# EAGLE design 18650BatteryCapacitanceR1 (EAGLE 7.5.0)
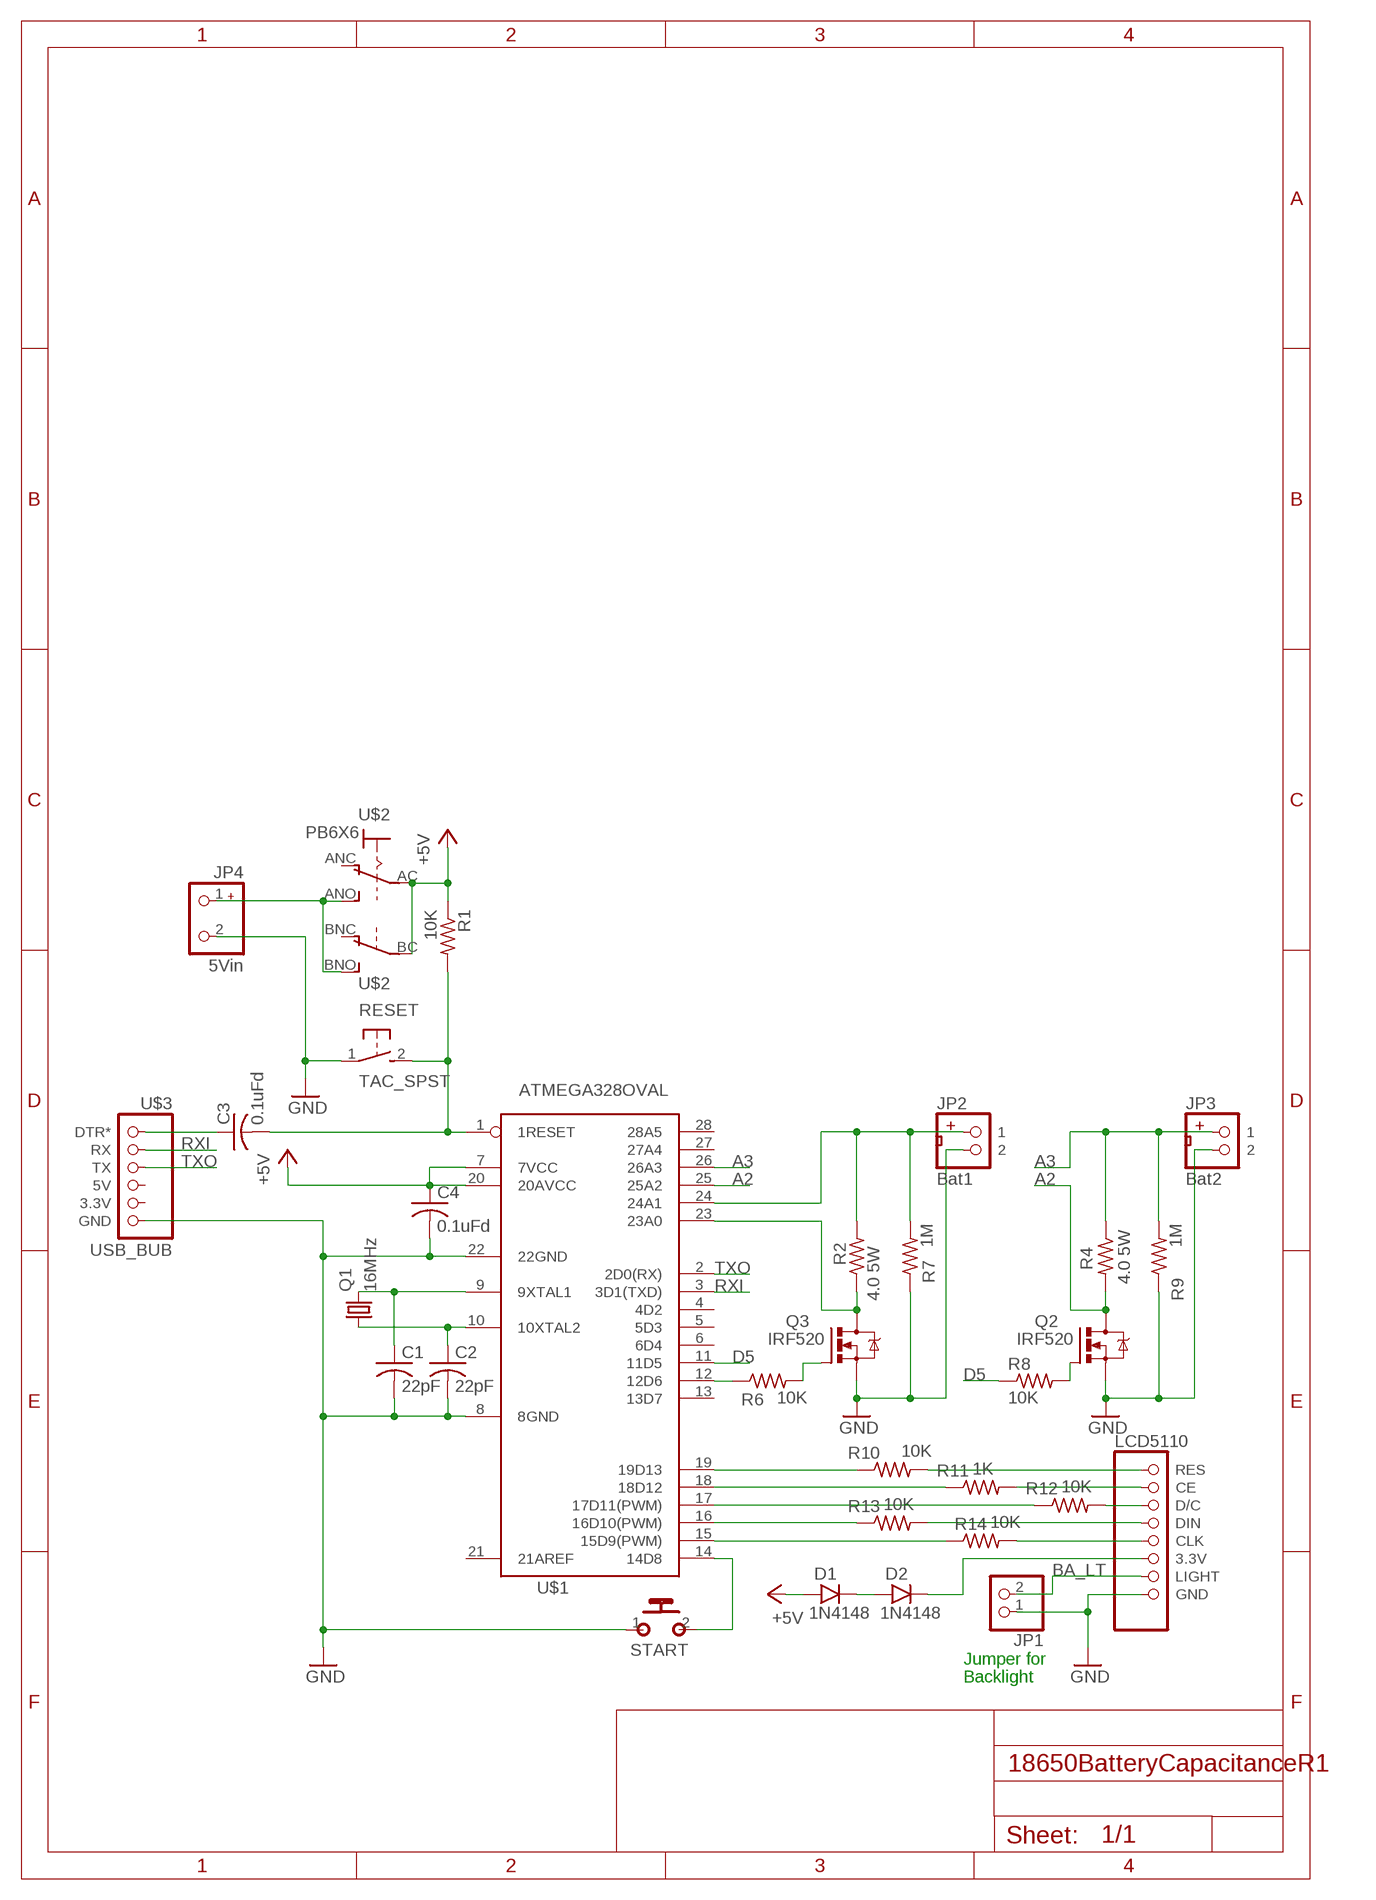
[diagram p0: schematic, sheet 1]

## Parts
C1  22pF  C-US025-025X050  [C025-025X050]
C2  22pF  C-US025-025X050  [C025-025X050]
C3  0.1uFd  C-US075-032X103  [C075-032X103]
C4  0.1uFd  C-US025-025X050  [C025-025X050]
D1  1N4148  1N4148-3  [DO35-3]
D2  1N4148  1N4148-3  [DO35-3]
JP1  PINHD-1X2  [1X02]
JP2  Bat1  JST2.0  [JST2.0]
JP3  Bat2  JST2.0  [JST2.0]
JP4  5Vin  KF301  [KF301]
LCD5110  LCD5110_1TOP  [LCD5110T1]
Q1  16MHz  CRYSTALHC49S  [HC49/S]
Q2  IRF520  [TO220BV]
Q3  IRF520  [TO220BV]
R1  10K  R-US_0207/7  [0207/7]
R2  4.0 5W  R-US_0922/22  [0922/22]
R4  4.0 5W  R-US_0922/22  [0922/22]
R6  10K  R-US_0207/7  [0207/7]
R7  1M  R-US_0207/2V  [0207/2V]
R8  10K  R-US_0207/7  [0207/7]
R9  1M  R-US_0207/2V  [0207/2V]
R10  10K  R-US_0207/2V  [0207/2V]
R11  1K  R-US_0207/2V  [0207/2V]
R12  10K  R-US_0207/2V  [0207/2V]
R13  10K  R-US_0207/2V  [0207/2V]
R14  10K  R-US_0207/2V  [0207/2V]
RESET  TAC_SPST  [TACTILE-SPST]
START  MOMENTARY  [SPST]
U$1  ATMEGA328OVAL  [DIL28-3]
U$2  PB6X6  [PB6X6]
U$3  USB_BUB  [USB_BUB]

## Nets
+5V: C4.1 D1.A R1.1 U$1.7(7VCC) U$1.20(20AVCC) U$2.AC(P) U$2.BC(P)
A2: Q2.D R4.2 U$1.25(25A2)
A3: JP3.1 R4.1 R9.2 U$1.26(26A3)
BA_LT: JP1.2 LCD5110.LIGHT
D5: R8.1 U$1.11(11D5)
GND: C1.2 C2.2 C4.2 JP1.1 JP2.2 JP3.2 JP4.2 LCD5110.GND Q2.S Q3.S R7.1 R9.1 RESET.1 START.1(P) U$1.8(8GND) U$1.22(22GND) U$3.GND
N$1: C1.1 Q1.2 U$1.9(9XTAL1)
N$2: C2.1 Q1.1 U$1.10(10XTAL2)
N$3: D2.C LCD5110.3.3V
N$4: JP4.1 U$2.ANO(S) U$2.BNO(S)
N$5: START.2(S) U$1.14(14D8)
N$6: C3.2 R1.2 RESET.2 U$1.1(1RESET)
N$7: C3.1 U$3.DTR*
N$8: Q2.G R8.2
N$9: D1.C D2.A
N$10: R10.1 U$1.19(19D13)
N$11: R11.1 U$1.18(18D12)
N$12: R12.1 U$1.17(17D11(PWM))
N$13: R13.1 U$1.16(16D10(PWM))
N$14: R14.1 U$1.15(15D9(PWM))
N$15: R6.1 U$1.12(12D6)
N$16: Q3.G R6.2
N$18: Q3.D R2.1 U$1.23(23A0)
N$20: JP2.1 R2.2 R7.2 U$1.24(24A1)
N$24: LCD5110.RES R10.2
N$25: LCD5110.CE R11.2
N$26: LCD5110.D/C R12.2
N$27: LCD5110.DIN R13.2
N$28: LCD5110.CLK R14.2
RXI: U$1.3(3D1(TXD)) U$3.RX
TXO: U$1.2(2D0(RX)) U$3.TX
Unconnected: U$1.4(4D2) U$1.5(5D3) U$1.6(6D4) U$1.13(13D7) U$1.21(21AREF) U$1.27(27A4) U$1.28(28A5) U$2.ANC(O) U$2.BNC(O) U$3.3.3V U$3.5V

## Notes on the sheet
- Jumper for
- Backlight

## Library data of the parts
C1-C4 = rcl:C-US: CAPACITOR, American symbol
D1 D2 = gm-diodes:1N4148: Fast Switching Diode
JP1 = pinhead:PINHD-1X2: PIN HEADER
JP2 JP3 = MTS_Custom:JST2.0
JP4 = MTS_Custom:KF301
LCD5110 = MTS_Custom:LCD5110_1
Q1 = crystal:CRYSTAL: CRYSTAL; OC_FARNELL: 1667008; OC_NEWARK: unknown
Q2 Q3 = transistor-power:IRF520: HEXFET Power MOSFET
R1 R6-R14 = rcl:R-US_: RESISTOR, American symbol
R2 R4 = resistor:R-US_: RESISTOR, American symbol
RESET = MTS_Custom:TAC_SPST: Tactile switch SPST 7mm lead spacing
START = MTS_Custom:MOMENTARY
U$1 = MTS_Custom:ATMEGA328
U$2 = MTS_Custom:PB6X6: Pushbutton 6mm x 6mm DPDT. should be the same for momentary and latching.
U$3 = MTS:USB_BUB

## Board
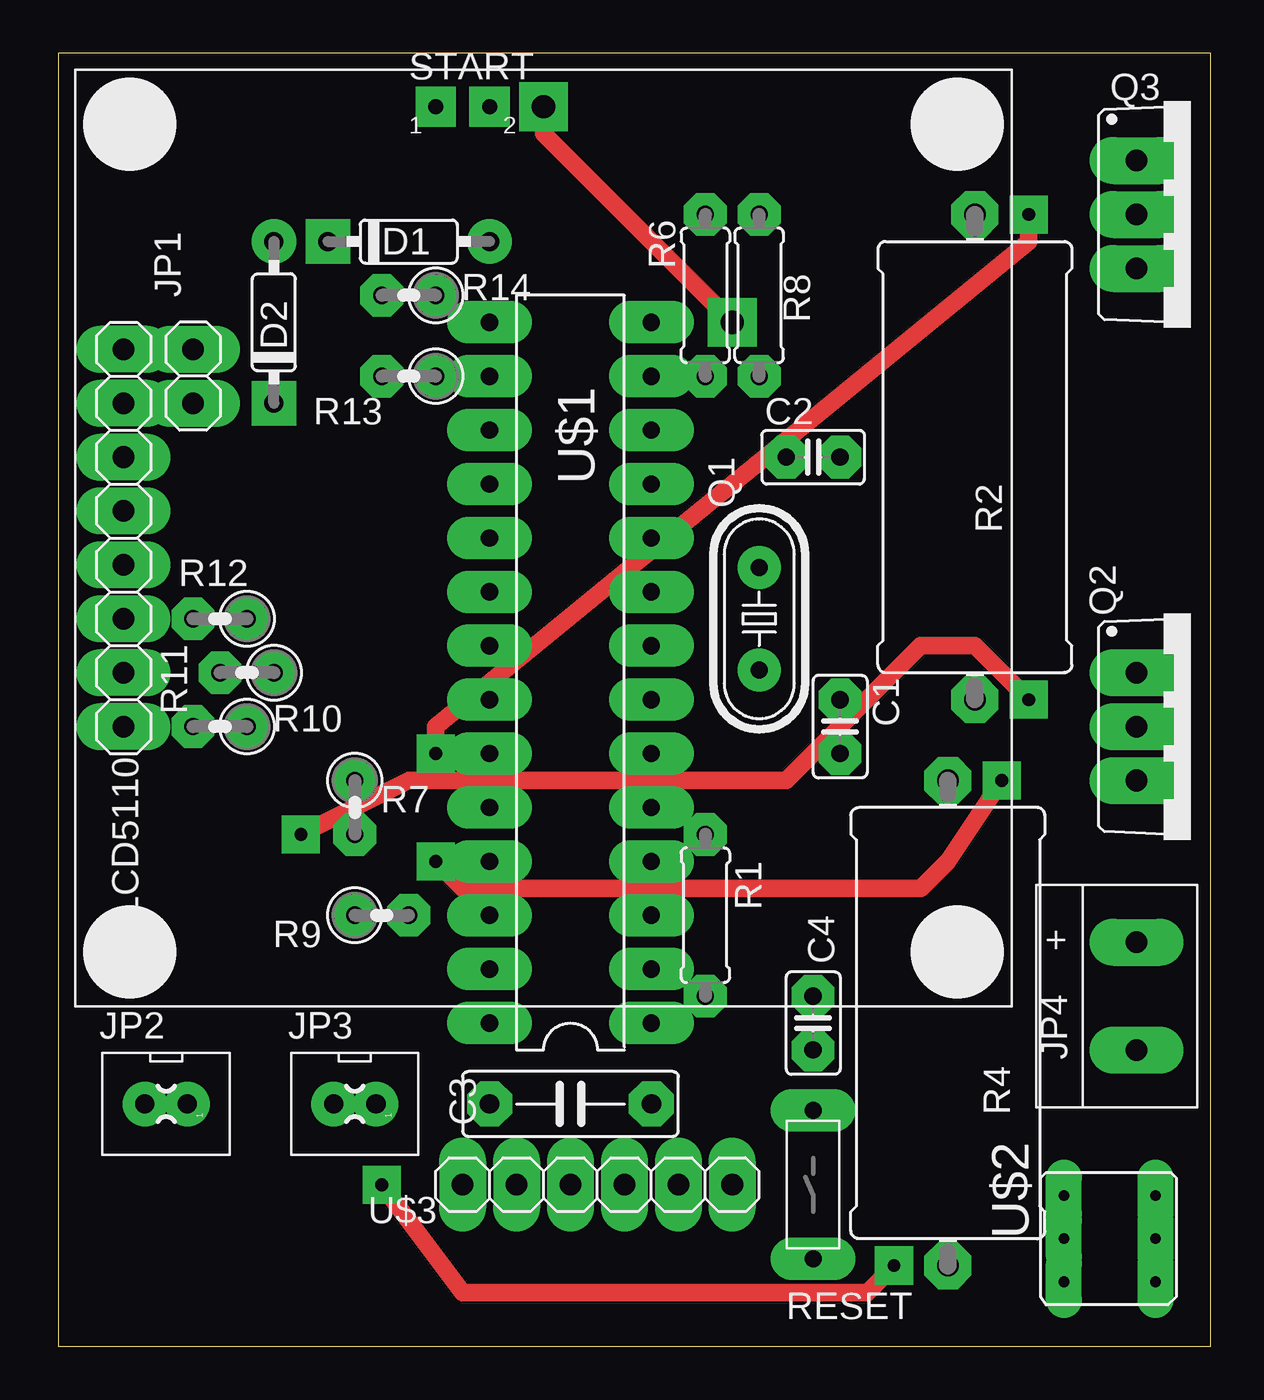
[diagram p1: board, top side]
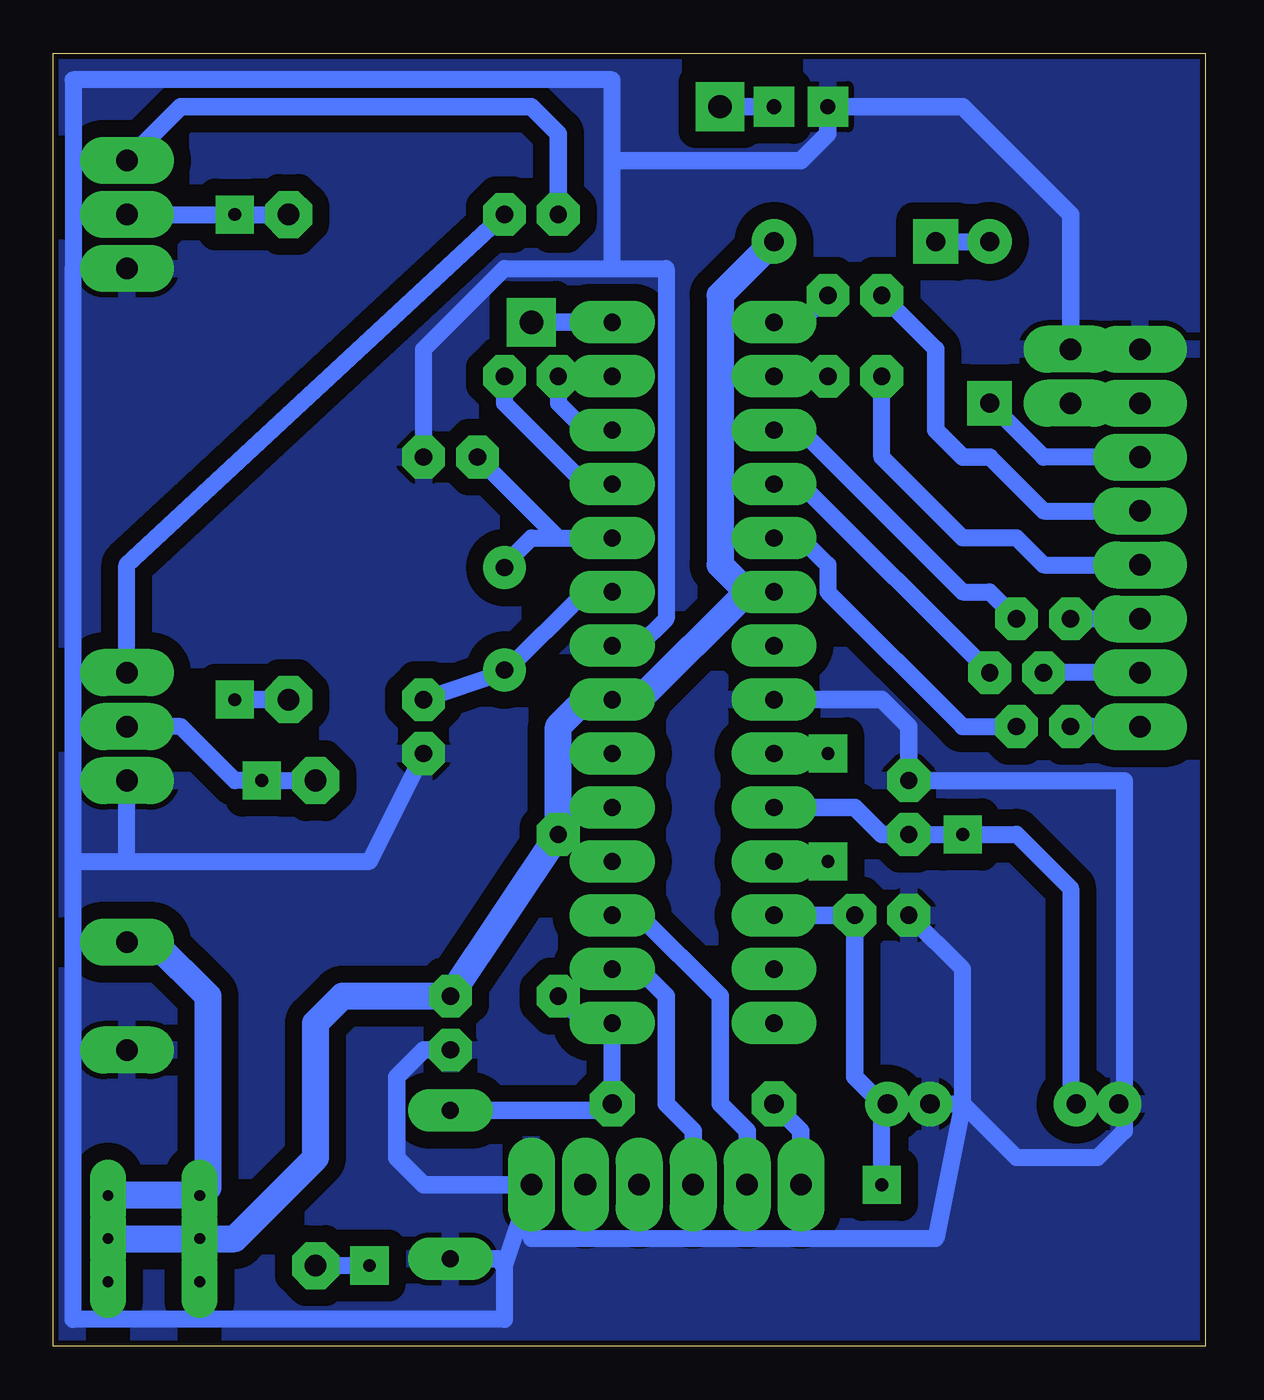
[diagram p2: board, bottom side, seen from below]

Size 54.28 x 60.95 mm. Coordinates in mm from the lower left corner, seen from the top.
Outline: 0,0 54.28,0 54.28,60.95 0,60.95 0,0
Copper layers (1*16): Top 0.035mm / dielectric 1.5mm / Bottom 0.035mm
Design rules "hobby": minimum track width 0.8mm, minimum drill 0.8mm, track to track 0.8mm, track to pad 0.8mm, pad to pad 0.45mm, via to via 0.8mm, smd to smd 8mil, copper to edge 10mil, drill to drill 8mil, minimum pad ring 0.6mm, minimum via ring 0.6mm, stop-mask expansion 0mil, vias tented up to drill 0mil, thermal gap 10mil

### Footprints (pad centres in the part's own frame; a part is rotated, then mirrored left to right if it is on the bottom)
C025-025X050 = drill 0.813 octagon: 1 -1.27,0; 2 1.27,0
C075-032X103 = drill 0.914 octagon: 1 -3.81,0; 2 3.81,0
DO35-3 = drill 0.9: A 3.81,0 | drill 0.9 square: C -3.81,0
1X02 = drill 1.016 long: 1 -1.27,0; 2 1.27,0
JST2.0 = drill 0.9 pad 1.016: 1 0,-1; 2 0,1
KF301 = drill 1.016 long: 1 -2.54,0; 2 2.54,0
LCD5110T1 = drill 1.016 long: 3.3V 3.81,19.78; CE -6.35,19.78; CLK 1.27,19.78; D/C -3.81,19.78; DIN -1.27,19.78; GND 8.89,19.78; LIGHT 6.35,19.78; RES -8.89,19.78
HC49/S = drill 0.813: 1 -2.413,0; 2 2.413,0
TO220BV = drill 1.016 long: D 0,-2.54; G -2.54,-2.54; S 2.54,-2.54
0207/7 = drill 0.813 octagon: 1 -3.81,0; 2 3.81,0
0922/22 = drill 1.016 octagon: 1 -11.43,0; 2 11.43,0
0207/2V = drill 0.813 octagon: 1 -1.27,0; 2 1.27,0
TACTILE-SPST = drill 0.8 long: 1 0,3.5; 2 0,-3.5
SPST = drill 0.7 square: 1 -1.27,0; 2 1.27,0
DIL28-3 = drill 0.813 long: 1 -16.51,-3.81; 2 -13.97,-3.81; 3 -11.43,-3.81; 4 -8.89,-3.81; 5 -6.35,-3.81; 6 -3.81,-3.81; 7 -1.27,-3.81; 8 1.27,-3.81; 9 3.81,-3.81; 10 6.35,-3.81; 11 8.89,-3.81; 12 11.43,-3.81; 13 13.97,-3.81; 14 16.51,-3.81; 15 16.51,3.81; 16 13.97,3.81; 17 11.43,3.81; 18 8.89,3.81; 19 6.35,3.81; 20 3.81,3.81; 21 1.27,3.81; 22 -1.27,3.81; 23 -3.81,3.81; 24 -6.35,3.81; 25 -8.89,3.81; 26 -11.43,3.81; 27 -13.97,3.81; 28 -16.51,3.81
PB6X6 = drill 0.5 pad 0.813 long: AC -2.159,0; ANC -2.159,-2.032; ANO -2.159,2.032; BC 2.159,0; BNC 2.159,-2.032; BNO 2.159,2.032
USB_BUB = drill 1.016 long: 3.3V -3.81,0; 5V -1.27,0; DTR* 6.35,0; GND -6.35,0; RX 3.81,0; TX 1.27,0

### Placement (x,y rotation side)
C1  36.83,29.21 270 top
C2  35.56,41.91 0 top
C3  24.13,11.43 0 top
C4  35.56,15.24 270 top
D1  16.51,52.07 0 top
D2  10.16,48.26 90 top
JP1  6.35,45.72 270 top
JP2  5.08,11.43 90 top
JP3  13.97,11.43 90 top
JP4  50.8,16.51 270 top
LCD5110  22.86,38.1 90 top
Q1  33.02,34.29 270 top
Q2  53.34,29.21 270 top
Q3  53.34,53.34 270 top
R1  30.48,20.32 270 top
R2  43.18,41.91 270 top
R4  41.91,15.24 90 top
R6  30.48,49.53 90 top
R7  13.97,25.4 270 top
R8  33.02,49.53 90 top
R9  15.24,20.32 0 top
R10  7.62,29.21 180 top
R11  8.89,31.75 180 top
R12  7.62,34.29 180 top
R13  16.51,45.72 180 top
R14  16.51,49.53 180 top
RESET  35.56,7.62 180 top
START  19.05,58.42 0 top
U$1  24.13,31.75 90 top
U$2  49.53,5.08 0 top
U$3  25.4,7.62 180 top

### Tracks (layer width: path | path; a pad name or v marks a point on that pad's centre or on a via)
+5V
  Bottom 1.27: 21.59,35.56 U$1.20 | 21.59,35.56 26.67,30.48 U$1.7 29.21,30.48 30.48,29.21 R1.1 C4.1 40.64,16.51 41.91,15.24 41.91,8.89 45.72,5.08 U$2.AC U$2.BC | D1.A 22.86,49.53 22.86,36.83 21.59,35.56
A2  (via drill 0.6)
  Top 0.813: v17.78,22.86 19.05,21.59 40.64,21.59 41.91,22.86 v44.45,26.67
  Bottom 0.8: R4.2 v44.45,26.67 45.72,26.67 48.26,29.21 Q2.D
  Bottom 0.813: U$1.25 v17.78,22.86
A3  (via drill 0.6)
  Top 0.813: v15.24,7.62 19.05,2.54 38.1,2.54 v39.37,3.81
  Bottom 0.8: v15.24,7.62 15.24,11.43 | v39.37,3.81 R4.1
  Bottom 0.813: U$1.26 R9.2 16.51,12.7 15.24,11.43 JP3.1
BA_LT
  Bottom 0.8: JP1.2 LCD5110.LIGHT
D5
  Bottom 0.8: U$1.11 29.21,40.64 33.02,44.45 R8.1
GND
  Bottom 0.8: JP1.1 LCD5110.GND | U$1.8 26.67,33.02 25.4,34.29 25.4,50.8 27.94,50.8 | 27.94,50.8 33.02,50.8 36.83,46.99 C2.2 | 53.34,50.8 53.34,59.69 27.94,59.69 27.94,55.88 27.94,50.8 | 3.81,11.43 3.81,26.67 R7.1 | R9.1 11.43,17.78 11.43,11.43 | JP3.2 11.43,11.43 | 11.43,11.43 8.89,8.89 5.08,8.89 3.81,10.16 3.81,11.43 | 3.81,11.43 JP2.2 | 11.43,11.43 12.7,5.08 31.75,5.08 U$3.GND 33.02,3.81 33.02,1.27 53.34,1.27 53.34,13.97 | 53.34,50.8 Q3.S | 53.34,13.97 53.34,22.86 | 53.34,22.86 53.34,50.8 | 53.34,13.97 JP4.2 | C1.2 39.37,22.86 50.8,22.86 | 53.34,22.86 50.8,22.86 | 50.8,22.86 Q2.S
  Bottom 0.813: R7.1 13.97,29.21 15.24,30.48 U$1.22 | RESET.1 33.33,4.12 33.02,3.81 | C4.2 36.83,13.97 38.1,12.7 38.1,8.89 36.83,7.62 U$3.GND | JP1.1 6.35,53.34 11.43,58.42 START.1 17.78,57.15 19.05,55.88 27.94,55.88
  pour Bottom: 0,0 54.61,0 54.61,60.96 0,60.96
N$1
  Bottom 0.8: 33.02,31.75 C1.1 | U$1.9 29.21,35.56 33.02,31.75 | 33.02,31.75 Q1.2
N$2
  Bottom 0.8: 30.48,38.1 31.75,38.1 33.02,36.83 Q1.1 | 30.48,38.1 U$1.10 | 30.48,38.1 C2.1
N$3
  Bottom 0.8: D2.C 7.62,41.91 LCD5110.3.3V
N$4
  Bottom 1.27: JP4.1 49.53,19.05 46.99,16.51 46.99,7.49 U$2.ANO U$2.BNO
N$5  (via drill 1.1)
  Top 0.813: v22.86,58.42 22.86,57.15 v31.75,48.26
  Bottom 0.813: START.2 v22.86,58.42 | v31.75,48.26 U$1.14
N$6
  Bottom 0.8: C3.2 U$1.1 29.21,15.24 R1.2
  Bottom 0.813: RESET.2 28.25,11.12 C3.2
N$7
  Bottom 0.813: C3.1 19.05,10.16 U$3.DTR*
N$8
  Bottom 0.8: R8.2 50.8,36.83 Q2.G
N$9
  Bottom 0.8: D1.C D2.A
N$10
  Bottom 0.8: R10.1 11.43,29.21 17.78,35.56 17.78,36.83 19.05,38.1 U$1.19
N$11
  Bottom 0.8: R11.1 19.05,40.64 U$1.18
N$12
  Bottom 0.8: R12.1 10.16,35.56 11.43,35.56 19.05,43.18 U$1.17
N$13
  Bottom 0.8: U$1.16 R13.1
N$14
  Bottom 0.8: R14.1 19.05,48.26 U$1.15
N$15
  Bottom 0.8: U$1.12 29.21,43.18 30.48,44.45 R6.1
N$16
  Bottom 0.813: Q3.G 48.26,58.42 31.75,58.42 30.48,57.15 R6.2
N$18  (via drill 0.6)
  Top 0.813: v17.78,27.94 17.78,29.21 45.72,52.07 v45.72,53.34
  Bottom 0.8: R2.1 v45.72,53.34 Q3.D
  Bottom 0.813: U$1.23 v17.78,27.94
N$20  (via drill 0.6)
  Top 0.813: v45.72,30.48 43.18,33.02 40.64,33.02 34.29,26.67 16.51,26.67 v11.43,24.13
  Bottom 0.8: JP2.1 6.35,11.43 6.35,21.59 8.89,24.13 v11.43,24.13 R7.2
  Bottom 0.813: U$1.24 16.51,25.4 15.24,24.13 R7.2 | R2.2 v45.72,30.48
N$24
  Bottom 0.8: LCD5110.RES R10.2
N$25
  Bottom 0.8: LCD5110.CE R11.2
N$26
  Bottom 0.8: LCD5110.D/C R12.2
N$27
  Bottom 0.8: R13.2 15.24,41.91 11.43,38.1 8.89,38.1 7.62,36.83 LCD5110.DIN
N$28
  Bottom 0.8: 12.7,46.99 R14.2 | 10.16,41.91 7.62,39.37 LCD5110.CLK
  Bottom 0.813: 12.7,46.99 12.7,43.18 11.43,41.91 10.16,41.91
RXI
  Bottom 0.813: U$3.RX 21.59,10.16 22.86,11.43 22.86,16.51 26.67,20.32 U$1.3
TXO
  Bottom 0.813: U$1.2 26.67,17.78 25.4,16.51 25.4,11.43 24.13,10.16 U$3.TX

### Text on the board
tValues: L.O.G. | + | + | + | + | 18650 Capacitance
bValues: Battery Capacitance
